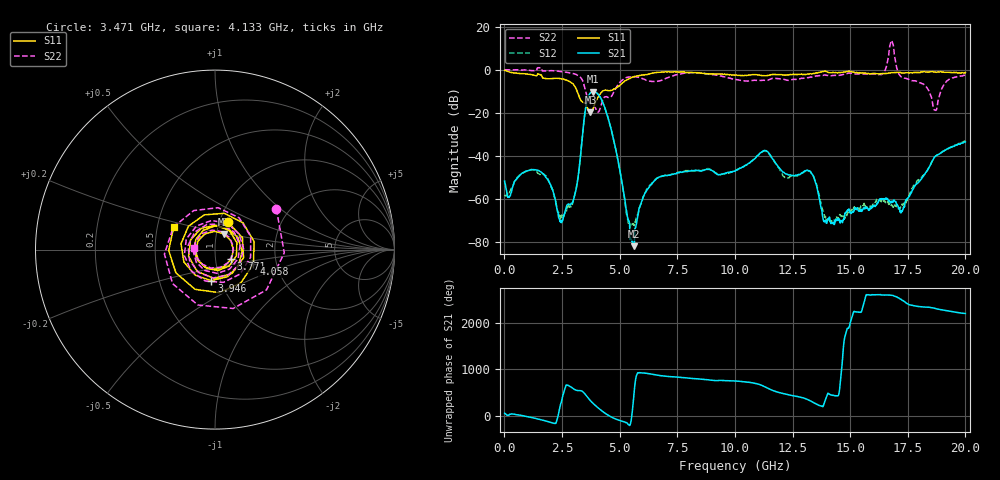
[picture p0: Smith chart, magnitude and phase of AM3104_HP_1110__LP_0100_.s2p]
!Created with skrf (http://scikit-rf.org).
# Hz S RI R 50.0
!freq ReS11 ImS11 ReS21 ImS21 ReS12 ImS12 ReS22 ImS22
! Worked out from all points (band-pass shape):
!   1601 points, 10 MHz to 20 GHz, reference 50 ohm
!   highest |S21| = -10.25 dB at 3.846 GHz (marker M1); lowest = -82.0 dB at 5.632 GHz (marker M2)
!   |S21| within 3 dB of the highest: 3.617 GHz to 4.183 GHz (565.6 MHz wide, 14.5 % of centre)
!   lowest |S11| = -19.9 dB at 3.733 GHz (marker M3), VSWR 1.22, Z = 54.5 + j9.58 ohm
!   |S11| at or under -10 dB: 3.151 GHz to 4.261 GHz (1.109 GHz wide, 29.9 % of centre)
!   |S22| runs from -19.8 to 13.5 dB; largest |S21 - S12| = 0.017
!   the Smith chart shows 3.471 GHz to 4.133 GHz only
!   S11 on the Smith chart (normalised r, x): 3.471 GHz: 1.10, +0.34; 3.771 GHz: 1.19, -0.13; 3.946 GHz: 0.91, -0.32; 4.058 GHz: 1.52, -0.26; 4.133 GHz: 0.61, +0.16
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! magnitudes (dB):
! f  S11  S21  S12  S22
! 10 MHz  -0.4  -51.8  -58.3  -0.1
! 1.309 GHz  -2.7  -46.5  -46.6  -0.6
! 2.471 GHz  -4.3  -71.1  -68.4  -0.9
! 2.996 GHz  -6.9  -60.5  -60.4  -1.8
! 3.346 GHz  -14.6  -35.2  -35.3  -4.2
! 3.471 GHz  -15.5  -22.1  -22.1  -7.8
! 3.733 GHz  -19.9  -10.8  -10.9  -15.9
! 3.771 GHz  -19.6  -10.5  -10.6  -15.9
! 3.846 GHz  -18.3  -10.2  -10.3  -16.5
! 3.946 GHz  -15.2  -10.5  -10.5  -17.7
! 4.058 GHz  -12.8  -11.4  -11.4  -19.7
! 4.133 GHz  -11.6  -12.4  -12.5  -18.7
! 5.632 GHz  -3.2  -82.0  -72.3  -3.4
! 6.682 GHz  -1.2  -50.1  -50.1  -5.4
! 10.01 GHz  -2.7  -47.2  -46.9  -4.6
! 11.3 GHz  -2.9  -37.6  -37.9  -5.0
! 13.34 GHz  -2.0  -48.5  -48.5  -3.4
! 13.93 GHz  -0.8  -70.2  -68.2  -2.5
! 16.68 GHz  -1.6  -61.4  -62.7  7.1
! 17.26 GHz  -1.5  -65.7  -62.7  -3.5
! 18.69 GHz  -1.2  -40.3  -40.3  -18.8
! 20 GHz  -1.4  -33.6  -33.1  -2.6
